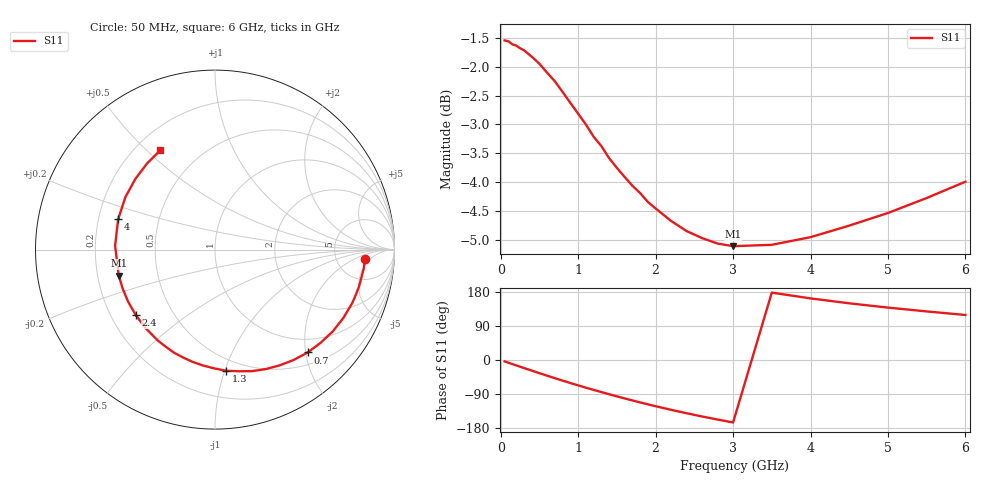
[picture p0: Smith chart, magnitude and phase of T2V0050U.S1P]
! SIEMENS Discrete & RF Semiconductors
! BAS70-04W
! Si Schottky Diode in SOT323
! IF = 0.05 mA
! S-Parameters:  November  1997
# GHz  S  MA  R  50
!  f  S11
! GHz  MAG  ANG
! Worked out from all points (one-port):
!   34 points, 50 MHz to 6 GHz, reference 50 ohm
!   lowest |S11| = -5.1 dB at 3 GHz (marker M1), VSWR 3.50, Z = 14.5 - j6.08 ohm
!   |S11| at or under -10 dB: nowhere
!   S11 on the Smith chart (normalised r, x): 50 MHz: 10, -4; 700 MHz: 0.72, -2.04; 1.3 GHz: 0.40, -1.01; 2.4 GHz: 0.30, -0.33; 4 GHz: 0.28, +0.14; 6 GHz: 0.30, +0.55
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0.05  0.8369 -3.7
0.1  0.8355 -7.2
0.2  0.8284 -14.3
0.3  0.8207 -21.2
0.4  0.8103 -28.0
0.5  0.7988 -34.8
0.6  0.7847 -41.5
0.7  0.7713 -48.0
0.8  0.7551 -54.5
0.9  0.7389 -60.8
1  0.7232 -67.0
1.1  0.7078 -73.1
1.3  0.678 -84.7
1.5  0.6492 -95.9
1.6  0.6376 -101.4
1.8  0.6175 -111.9
2  0.5988 -122.0
2.2  0.5841 -131.5
2.4  0.5724 -140.5
2.6  0.5645 -149.1
2.8  0.5584 -157.1
3  0.5555 -164.9
3.5  0.557 177.8
4  0.5655 162.6
4.5  0.5787 149.6
5  0.5935 138.3
5.5  0.6114 128.2
6  0.6316 118.8
